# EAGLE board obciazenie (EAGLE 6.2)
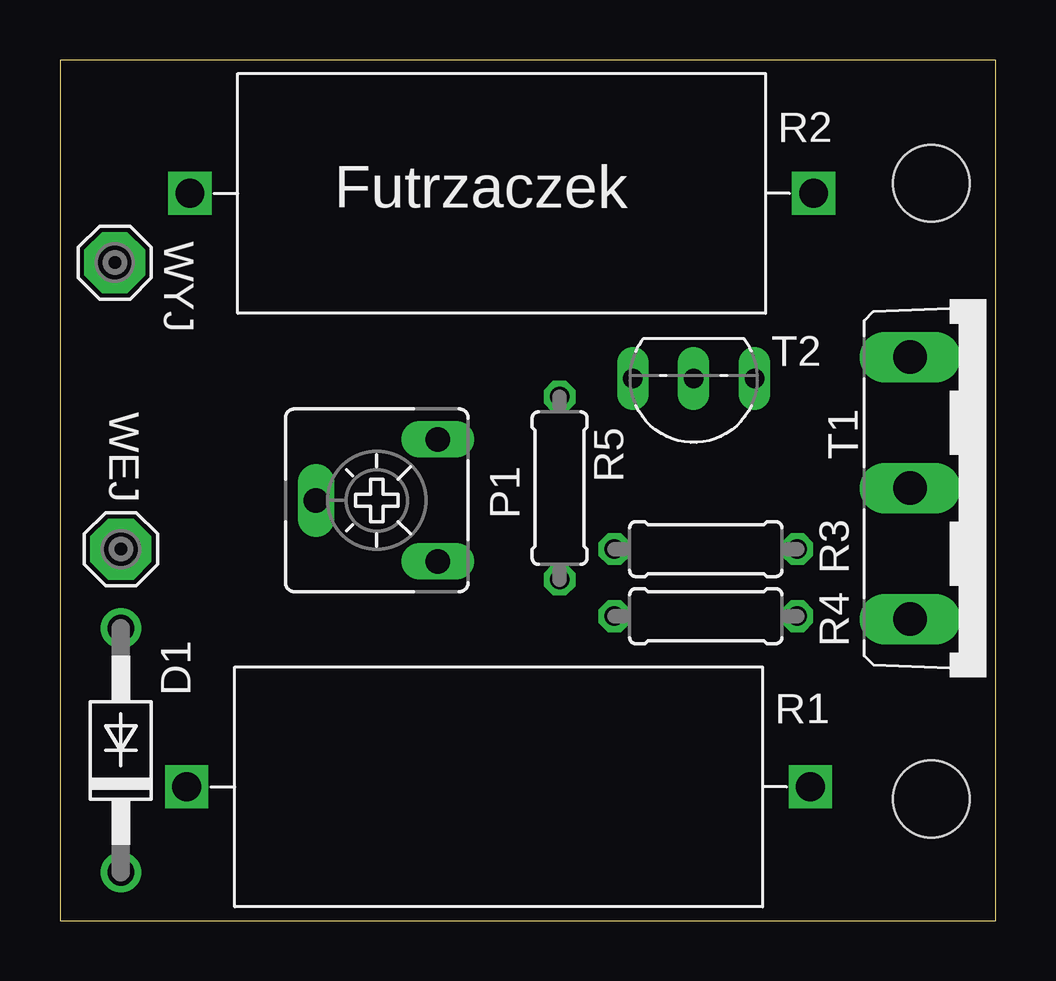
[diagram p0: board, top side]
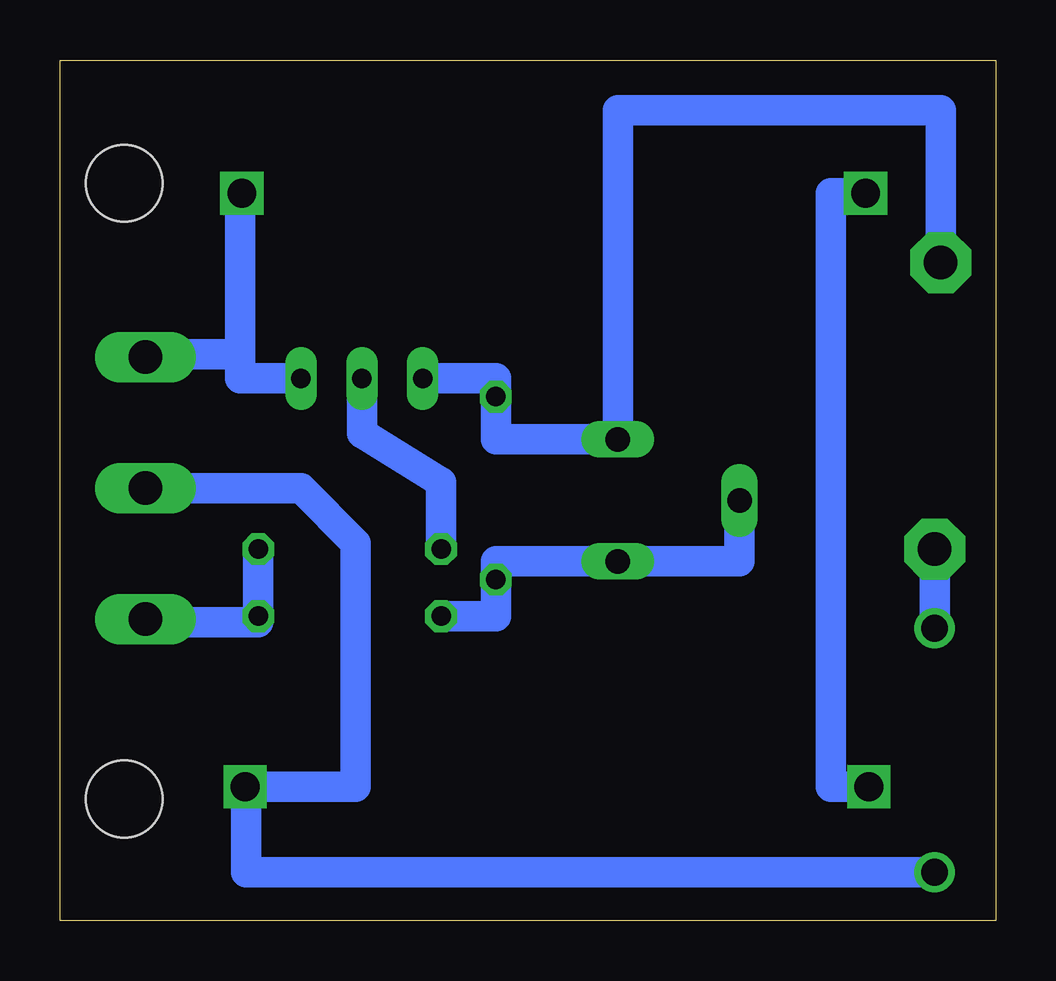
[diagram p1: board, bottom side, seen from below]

Size 39 x 35.87 mm. Coordinates in mm from the lower left corner, seen from the top.
Outline: 0,0 39,0 39,35.87 0,35.87 0,0
Copper layers (1*16): Top 0.035mm / dielectric 1.5mm / Bottom 0.035mm
Design rules: minimum track width 10mil, minimum drill 24mil, track to track 8mil, track to pad 8mil, pad to pad 8mil, via to via 8mil, smd to smd 8mil, copper to edge 40mil, drill to drill 8mil, minimum pad ring 10mil, minimum via ring 8mil, stop-mask expansion 4mil, vias tented up to drill 0mil, thermal gap 10mil
Holes 3.2 mm at 36.32,5.08 36.32,30.73

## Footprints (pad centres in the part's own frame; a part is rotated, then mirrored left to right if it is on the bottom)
DO41-10 = drill 1.118: A 5.08,0; C -5.08,0
CA6V = drill 1.016 long: A -2.54,-2.54; E 2.54,-2.54; S 0,2.54
R_5W = drill 1.2 square: P$1 -13,0; P$2 13,0
0207/7 = drill 0.813 octagon: 1 -3.81,0; 2 3.81,0
TOP3V = drill 1.397 long: B -5.461,-3.175; C 0,-3.175; E 5.461,-3.175
TO92-EBC = drill 0.813 long: B 0,-1.27; C -2.54,-1.27; E 2.54,-1.27
SE14 = drill 1.397 pad 2.54 octagon: MP 0,0

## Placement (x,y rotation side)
D1  1N4007  [DO41-10]  2.54,7.11 90 top
P1  100  [CA6V]  13.21,17.53 90 top
R1  47k/5W  [R_5W]  18.28,5.59 0 top
R2  47k/5W  [R_5W]  18.42,30.32 180 top
R3  1k  [0207/7]  26.92,15.49 180 top
R4  10  [0207/7]  26.92,12.7 0 top
R5  120  [0207/7]  20.83,18.03 270 top
T1  2SC5129  [TOP3V]  38.61,18.03 270 top
T2  BC337  [TO92-EBC]  26.42,21.34 180 top
WEJ  SE14  [SE14]  2.54,15.49 0 top
WYJ  SE14  [SE14]  2.29,27.43 0 top

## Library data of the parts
D1 = diode
P1 = pot
R1 R2 T1 = inne_futrzak
R3-R5 = rcl
T2 = transistor-npn
WEJ WYJ = solpad

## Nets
N$1: R1.P$1 R2.P$2
N$2: R2.P$1 T1.B T2.C
N$3: R3.2 T2.B
N$4: R3.1 R4.2 T1.E
N$5: P1.A P1.S R4.1 R5.2
N$7: D1.A WEJ.MP
N$8: P1.E R5.1 T2.E WYJ.MP
N$9: D1.C R1.P$2 T1.C

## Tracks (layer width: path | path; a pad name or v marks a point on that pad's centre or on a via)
N$1
  Bottom 1.27: R2.P$2 6.86,30.32 6.86,5.59 R1.P$1
N$2
  Bottom 1.27: 31.5,23.62 31.5,30.23 31.42,30.23 R2.P$1 | 31.5,23.62 35.43,23.62 T1.B | T2.C 31.5,22.61 31.5,23.62
N$3
  Bottom 1.27: R3.2 23.11,18.29 26.42,20.32 T2.B
N$4
  Bottom 1.27: R3.1 R4.2 30.73,12.45 35.43,12.45 T1.E
N$5
  Bottom 1.27: P1.S 10.67,14.99 P1.A 20.83,14.99 R5.2 20.83,12.7 R4.1
N$7
  Bottom 1.27: WEJ.MP D1.A
N$8
  Bottom 1.27: WYJ.MP 2.29,33.78 15.75,33.78 P1.E 20.83,20.07 R5.1 20.83,22.61 T2.E
N$9
  Bottom 1.27: D1.C 31.24,2.03 31.24,5.59 | 31.24,5.59 26.67,5.59 26.67,15.75 28.96,18.03 T1.C | 31.24,5.59 R1.P$2

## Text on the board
tPlace: Futrzaczek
